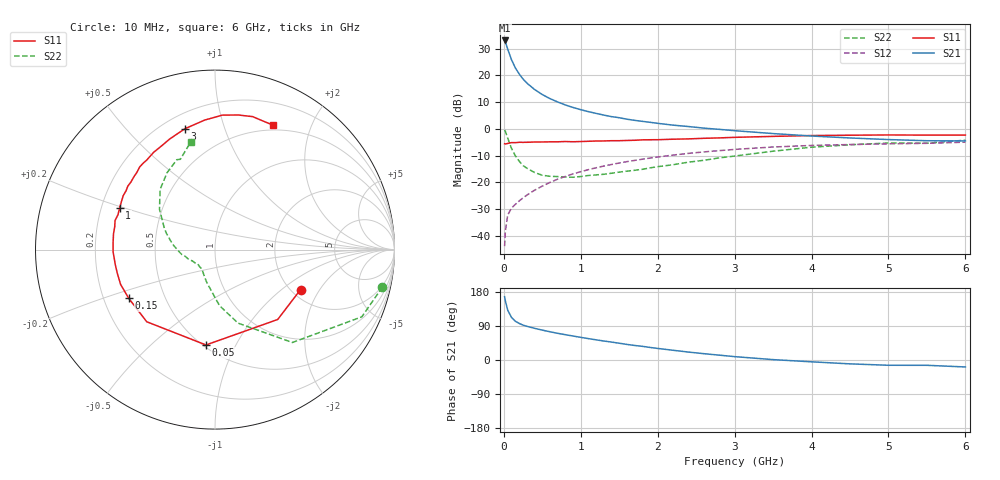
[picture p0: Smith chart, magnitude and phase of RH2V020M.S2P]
! SIEMENS Small Signal Semiconductors
! BFR106
! Si NPN RF Bipolar Junction Transistor in SOT23
! VCE = 2 V  IC = 20 mA
! Common Emitter S-Parameters:  August  1996
# GHz  S  MA  R  50
!  f  S11  S21  S12  S22
! GHz  MAG  ANG  MAG  ANG  MAG  ANG  MAG  ANG
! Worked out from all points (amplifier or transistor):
!   36 points, 10 MHz to 6 GHz, reference 50 ohm
!   highest |S21| = 33.1 dB at 10 MHz (marker M1)
!   |S21| within 3 dB of that: start of sweep to 47.74 MHz
!   unconditionally stable (mu >= 1): 356.4 MHz to 2.538 GHz; 5.001 GHz to end of sweep
!   at 250 MHz: K = 0.90, MSG = 22.2 dB, |S12| = -25.8 dB
!   at 1.4 GHz: K = 1.08, MAG = 7.2 dB, |S12| = -13.3 dB
!   at 6 GHz: K = 1.01, MAG = -0.5 dB, |S12| = -5.0 dB
!   S11 on the Smith chart (normalised r, x): 10 MHz: 2.24, -1.38; 50 MHz: 0.52, -0.77; 150 MHz: 0.31, -0.24; 1 GHz: 0.28, +0.19; 3 GHz: 0.29, +0.74; 6 GHz: 0.44, +1.48
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0.01  0.5262 -25.0  45.06 166.9  0.0064 81.4  0.9559 -12.6
0.02  0.5231 -48.1  42.37 155.9  0.0123 71.9  0.8997 -24.6
0.05  0.5337 -95.4  31.17 131.6  0.0243 56.7  0.6737 -50.2
0.1  0.5534 -133.4  19.59 112.2  0.0331 49.9  0.4293 -72.6
0.15  0.552 -150.5  13.77 102.2  0.0388 51.6  0.3134 -85.4
0.2  0.5607 -159.8  10.62 96.5  0.045 54.1  0.2481 -92.4
0.25  0.56 -166.4  8.547 92.0  0.0512 56.1  0.2059 -99.8
0.3  0.5615 -170.9  7.177 88.9  0.0578 59.1  0.1838 -105.2
0.4  0.5678 -178.6  5.448 83.6  0.0713 62.0  0.1526 -114.2
0.5  0.569 176.3  4.381 78.8  0.085 63.1  0.1356 -121.2
0.6  0.5723 171.2  3.682 74.5  0.0997 64.0  0.1298 -126.3
0.8  0.5799 163.8  2.8 66.8  0.1292 63.8  0.1259 -136.7
1  0.58 156.3  2.285 59.8  0.1582 62.5  0.1286 -143.0
1.1  0.5859 152.9  2.099 56.4  0.1731 61.7  0.1344 -146.9
1.3  0.5941 146.5  1.809 50.1  0.2017 59.2  0.1416 -153.8
1.6  0.6072 138.1  1.517 41.1  0.244 55.4  0.162 -162.8
2.2  0.6408 122.2  1.174 25.7  0.3236 46.5  0.2134 179.1
3  0.6943 103.8  0.925 8.9  0.413 33.7  0.3103 156.2
3.5  0.7238 94.6  0.817 1.0  0.4578 26.0  0.3824 144.0
4.5  0.7611 80.2  0.676 -10.2  0.5095 11.0  0.5044 122.0
5.5  0.7643 68.5  0.6 -14.0  0.5373 1.7  0.5389 111.0
6  0.7655 64.9  0.595 -18.4  0.5639 -5.3  0.6149 102.7
